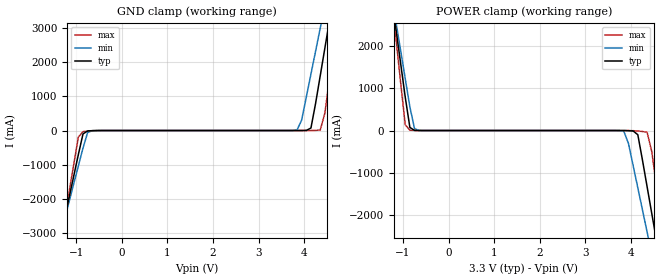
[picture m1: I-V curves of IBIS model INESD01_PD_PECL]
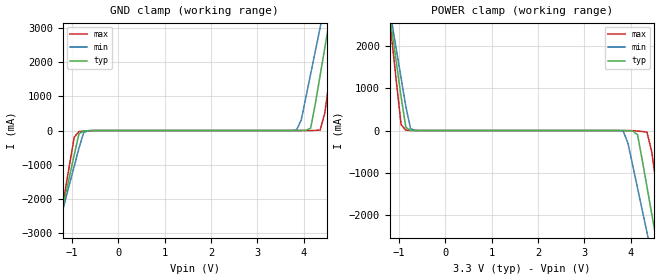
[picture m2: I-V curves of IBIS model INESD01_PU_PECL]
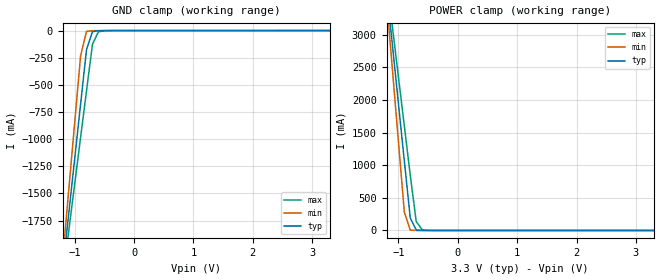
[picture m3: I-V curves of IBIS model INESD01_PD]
|   This file is an IBIS representation of the   |
|   Integrated Device Technology , Inc.   |
|   ICS8531-01   |
|   Low Skew 1 to 9 Differential to 3.3V LVPECL Clock Buffer   |
[IBIS Ver]   4.1
[File name]   8531_01_3v3.ibs
[File Rev]   3.0
[Date]   31 Aug 2009 | Last modified
|   Apr 5 2005 | Generated
[Source]   Originated at Integrated Device Technology, Inc.
[Disclaimer]
IDT hereby grants the user of this IBIS model a non-exclusive,
nontransferable license to use this IBIS model under the following terms.
Before using this IBIS model, the user should read this license.
If the user does not accept these terms,  the IBIS model should be
returned to IDT within 30 days.
   The user is granted this license only to use the IBIS model and
is not granted rights to sell, load, rent, lease or license the IBIS
model in whole or in part, or in modified form to anyone other than
user. User may modify the IBIS model to suit its specific
applications but rights to derivative works and such modifications
shall belong to IDT.
   This IBIS model is provided on an "AS IS" basis and IDT makes
absolutely no warranty with respect to the information contained
herein. IDT DISCLAIMS AND CUSTOMER WAIVES ALL WARRANTIES, EXPRESS
OR IMPLIED, INCLUDING WARRANTIES OF MERCHANTABILITY OR FITNESS FOR
A PARTICULAR PURPOSE. The entire risk as to quality and performance
is with the Customer. ACCORDINGLY, IN NO EVENT SHALL THE COMPANY BE
LIABLE FOR ANY DAMAGES, WHETHER IN CONTRACT OR TORT,INCLUDING ANY
LOST PROFITS OR OTHER INCIDENTAL, CONSEQUENTIAL, EXEMPLARY, OR
PUNITIVE DAMAGES ARISING OUT OF THE USE OR APPLICATION OF THE IBIS
model provided in this package. Further, IDT reserves the right to
make changes without notice to any product herein to improve
reliability, function, or design. IDT does not convey any license
under patent rights or any other intellectual property rights,
including those of third parties.
   IDT is not obligated to provide maintenance or support
for the licensed IBIS model.
[Copyright]   Copyright 2005 by Integrated Device Technology , Inc.
[Component]   ICS8531Y-01
[Manufacturer] Integrated Device Technology, Inc.
[Package]
|LQFP32
|lead + wire   typ   min   max
R_pkg   220.4m   212.5m   238m
L_pkg   1.841n   1.708n   1.974n
C_pkg   0.316p   0.2907p   0.33p
[Pin] signal_name   model_name   R_pin   L_pin   C_pin
1   VCC   POWER   238m   1.974n   0.330p
2   CLK   INESD01_PD_PECL   225m   1.841n   0.311p
3   nCLK   INESD01_PU_PECL   218m   1.7745n   0.301p
4   CLK_SEL   INESD01_PD   213m   1.708n   0.291p
5   PCLK   INESD01_PD_PECL   213m   1.708n   0.291p
6   nPCLK   INESD01_PU_PECL   218m   1.7745n   0.301p
7   VEE   GND   225m   1.841n   0.311p
8   CLK_EN   INESD01_PU   238m   1.974n   0.330p
9   VCCO   POWER   238m   1.974n   0.330p
10   nQ8   ONF01_PECL01_CBI   225m   1.841n   0.311p
11   Q8   ONF01_PECL01_CBI   218m   1.7745n   0.301p
12   nQ7   ONF01_PECL01_CBI   213m   1.708n   0.291p
13   Q7   ONF01_PECL01_CBI   213m   1.708n   0.291p
14   nQ6   ONF01_PECL01_CBI   218m   1.7745n   0.301p
15   Q6   ONF01_PECL01_CBI   225m   1.841n   0.311p
16   VCCO   POWER   238m   1.974n   0.330p
17   VCCO   POWER   238m   1.974n   0.330p
18   nQ5   ONF01_PECL01_CBI   225m   1.841n   0.311p
19   Q5   ONF01_PECL01_CBI   218m   1.7745n   0.301p
20   nQ4   ONF01_PECL01_CBI   213m   1.708n   0.291p
21   Q4   ONF01_PECL01_CBI   213m   1.708n   0.291p
22   nQ3   ONF01_PECL01_CBI   218m   1.7745n   0.301p
23   Q3   ONF01_PECL01_CBI   225m   1.841n   0.311p
24   VCCO   POWER   238m   1.974n   0.330p
25   VCCO   POWER   238m   1.974n   0.330p
26   nQ2   ONF01_PECL01_CBI   225m   1.841n   0.311p
27   Q2   ONF01_PECL01_CBI   218m   1.7745n   0.301p
28   nQ1   ONF01_PECL01_CBI   213m   1.708n   0.291p
29   Q1   ONF01_PECL01_CBI   213m   1.708n   0.291p
30   nQ0   ONF01_PECL01_CBI   218m   1.7745n   0.301p
31   Q0   ONF01_PECL01_CBI   225m   1.841n   0.311p
32   VCCO   POWER   238m   1.974n   0.330p
[Diff Pin]  inv_pin  vdiff tdelay_typ tdelay_min  tdelay_max
2   3   0.15   0   0   0
5   6   0.15   0   0   0
11   10   NA   0   0   0
13   12   NA   0   0   0
15   14   NA   0   0   0
19   18   NA   0   0   0
21   20   NA   0   0   0
23   22   NA   0   0   0
27   26   NA   0   0   0
29   28   NA   0   0   0
31   30   NA   0   0   0
| Models and submodels in the file (5): INESD01_PD_PECL (Input), INESD01_PU_PECL (Input), INESD01_PD (Input), INESD01_PU (Input), ONF01_PECL01_CBI (Output_ECL)
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[Model]   INESD01_PD_PECL
Model_type  Input
Polarity   Non-Inverting
Vinl = 0.8V
Vinh = 2.0V
|   typ   min   max
C_comp   2pF   1.5pF   2.5pF
|   typ   min   max
[Voltage range]  3.3V   3.15V   3.45V
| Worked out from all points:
|   GND clamp passes 1 mA (typ) near -0.55 V on its own axis
|   POWER clamp passes 1 mA (typ) near -0.66 V on its own axis
[GND_clamp]
|Voltage   I(typ)   I(min)   I(max)
-2.586V   -10.86A    -9.487A    -13.15A
-1.361V   -3.24A     -3.145A    -3.432A
-1.259V   -2.606A    -2.617A    -2.622A
-952.6mV  -705.3mA   -1.038A    -192.4mA
-850.5mV  -99.9mA    -513.5mA   -31.23mA
-646.4mV  -3.788mA   -3.549mA   -8.297mA
3.844V    129.1uA    13.13mA    71.12uA
4.151V    73.33mA    1.652A     864.7uA
4.355V    1.607A     3.003A     15.44mA
4.559V    3.233A     4.356A     1.553A
4.763V    4.861A     5.711A     3.635A
5.375V    9.757A     9.783A     9.893A
[POWER_clamp]
|Voltage   I(typ)   I(min)   I(max)
-2.177V   10.57A     9.364A     12.62A
-1.157V   2.42A      2.586A     2.194A
-952.6mV  795.8mA    1.237A     137.8mA
-850.5mV  73.33mA    563.2mA    8.145mA
-646.4mV  535.8uA    2.004mA    431.2uA
3.844V    -826.3uA   -18.14mA   -47.07uA
4.151V    -99.9mA    -1.362A    -11.82mA
4.355V    -1.338A    -2.415A    -41.71mA
4.559V    -2.606A    -3.47A     -1.312A
4.661V    -3.24A     -3.998A    -2.123A
4.763V    -3.875A    -4.526A    -2.933A
5.579V    -8.954A    -8.756A    -9.414A
[Model]   INESD01_PU_PECL
Model_type  Input
Polarity   Non-Inverting
Vinl = 0.8V
Vinh = 2.0V
|   typ   min   max
C_comp   2pF   1.5pF   2.5pF
|   typ   min   max
[Voltage range]  3.3V   3.15V   3.45V
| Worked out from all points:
|   GND clamp passes 1 mA (typ) near -0.55 V on its own axis
|   POWER clamp passes 1 mA (typ) near -0.67 V on its own axis
[GND_clamp]
|Voltage   I(typ)   I(min)   I(max)
-3.3V     -15.3A     -13.19A    -18.82A
-1.361V   -3.24A     -3.145A    -3.432A
-1.259V   -2.606A    -2.617A    -2.622A
-952.6mV  -705.4mA   -1.038A    -192.5mA
-850.5mV  -99.96mA   -513.6mA   -31.29mA
-646.4mV  -3.852mA   -3.611mA   -8.361mA
3.844V    64.83uA    13.07mA    7.183uA
4.151V    73.26mA    1.652A     800.8uA
4.355V    1.607A     3.003A     15.37mA
4.559V    3.233A     4.356A     1.553A
4.763V    4.861A     5.711A     3.635A
6.6V      19.56A     17.94A     22.42A
[POWER_clamp]
|Voltage   I(typ)   I(min)   I(max)
-3.3V     19.56A     16.84A     24.11A
-1.259V   3.233A     3.262A     3.235A
-1.157V   2.419A     2.586A     2.194A
-952.6mV  795.8mA    1.236A     137.7mA
-850.5mV  73.26mA    563.1mA    8.081mA
-646.4mV  471.5uA    1.942mA    367.2uA
3.844V    -890.5uA   -18.21mA   -111uA
4.151V    -99.96mA   -1.362A    -11.88mA
4.355V    -1.338A    -2.415A    -41.77mA
4.559V    -2.606A    -3.47A     -1.313A
4.763V    -3.875A    -4.526A    -2.933A
6.6V      -15.3A     -14.05A    -17.51A
[Model]   INESD01_PD
Model_type   Input
Polarity   Non-Inverting
Vinl = 0.80V
Vinh = 2.0V
|   typ   min   max
C_comp   2pF   1.5pF   2.5pF
|   typ   min   max
[Voltage range]  3.3V   3.15V   3.45V
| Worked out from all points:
|   GND clamp passes 1 mA (typ) near -0.55 V on its own axis
|   POWER clamp passes 1 mA (typ) near -0.60 V on its own axis
[GND_clamp]
|Voltage I(typ)   I(min)   I(max)
-3.3V     -12.83A    -15.14A    -11.37A
-1.2V     -2.195A    -2.092A    -2.281A
-1.1V     -1.689A    -1.472A    -1.849A
-900mV    -678.5mA   -232.6mA   -984.8mA
-800mV    -173.9mA   -7.175mA   -553.2mA
-700mV    -9.696mA   -1.052mA   -126mA
-600mV    -1.629mA   -178uA     -11.07mA
-300mV    -10.53uA   -5.678uA   -86.08uA
3.3V      71.13uA    62.11uA    77.58uA
[POWER_clamp]
|Voltage   I(typ)   I(min)   I(max)
-3.3V     22.38A     26.45A     19.82A
-1.2V     3.723A     3.545A     3.874A
-1.1V     2.836A     2.457A     3.116A
-1V       1.949A     1.369A     2.358A
-900mV    1.063A     281.1mA    1.601A
-800mV    191.6mA    5.074mA    844mA
-700mV    8.104mA    204.3uA    138.4mA
-600mV    678.1uA    79.74uA    10.7mA
-400mV    87.44uA    69.65uA    413.2uA
3.3V      -3.041nA   -425fA     -919.9nA
